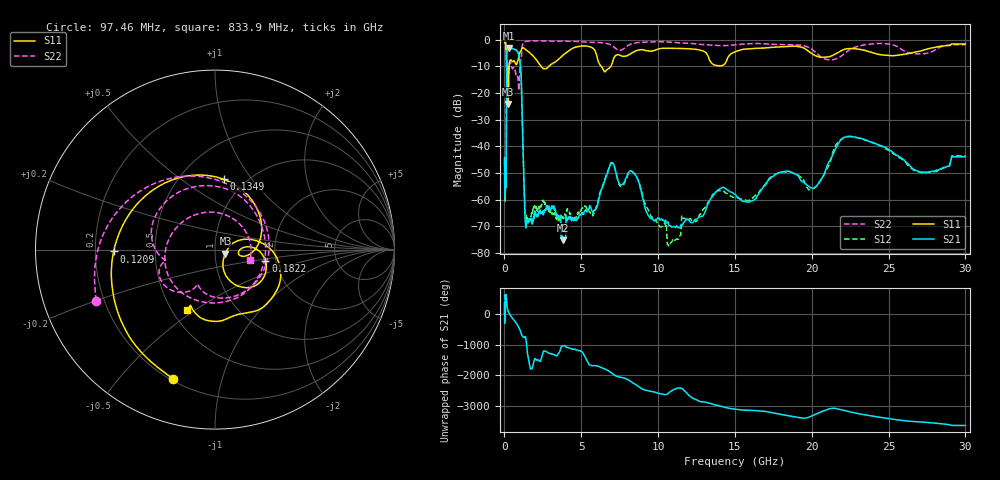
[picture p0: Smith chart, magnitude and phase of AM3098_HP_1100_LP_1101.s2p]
! Date/Time: Thu, Feb 28, 2019 8:44 AM
! Network Analyzer: Agilent Technologies E8364B Rev: A.07.50.67
! Sweep from 0.010 to 30.000 GHz, 1601 Points, Sweep Type: LOG
! Power Supply: 5.022 V, 0.002 A
# Hz S DB R 50
!freq MagS11 AngS11 MagS21 AngS21 MagS12 AngS12 MagS22 AngS22
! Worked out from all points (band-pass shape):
!   1601 points, 10 MHz to 30 GHz, reference 50 ohm
!   highest |S21| = -3.10 dB at 266.5 MHz (marker M1); lowest = -75.4 dB at 3.817 GHz (marker M2)
!   |S21| within 3 dB of the highest: 149.2 MHz to 943.7 MHz (794.5 MHz wide, 145 % of centre)
!   lowest |S11| = -24.1 dB at 248.4 MHz (marker M3), VSWR 1.13, Z = 56.1 - j2.53 ohm
!   |S11| at or under -10 dB: 140.1 MHz to 310.6 MHz (170.5 MHz wide, 75.6 % of centre); 2.372 GHz to 2.907 GHz (534.3 MHz wide, 20.2 % of centre); 6.291 GHz to 6.926 GHz (634.8 MHz wide, 9.61 % of centre)
!   |S22| runs from -19.1 to -0.4 dB; largest |S21 - S12| = 0.011
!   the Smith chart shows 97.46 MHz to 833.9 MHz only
!   S11 on the Smith chart (normalised r, x): 97.46 MHz: 0.21, -0.71; 120.9 MHz: 0.28, -0.01; 134.9 MHz: 0.80, +0.74; 182.2 MHz: 1.76, -0.23; 833.9 MHz: 0.59, -0.46
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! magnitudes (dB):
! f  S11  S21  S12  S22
! 10 MHz  -0.3  -46.6  -44.1  -0.6
! 38.04 MHz  -0.4  -57.1  -55.2  -0.9
! 97.46 MHz  -2.4  -54.4  -52.7  -2.9
! 120.9 MHz  -5.0  -36.3  -35.7  -6.4
! 134.9 MHz  -8.1  -14.7  -14.7  -10.5
! 144.7 MHz  -12.3  -7.5  -7.4  -11.7
! 182.2 MHz  -10.8  -3.9  -3.9  -9.8
! 248.4 MHz  -24.1  -3.1  -3.1  -11.0
! 266.5 MHz  -17.9  -3.1  -3.1  -10.7
! 550.5 MHz  -8.2  -3.5  -3.4  -10.8
! 833.9 MHz  -8.6  -4.4  -4.4  -13.9
! 1.071 GHz  -4.3  -12.0  -12.0  -7.7
! 1.375 GHz  -3.7  -69.9  -66.2  -0.7
! 2.084 GHz  -7.6  -66.0  -63.6  -0.5
! 3.172 GHz  -8.9  -62.8  -65.5  -0.6
! 3.817 GHz  -5.8  -75.4  -66.8  -0.5
! 7.926 GHz  -6.1  -51.7  -52.4  -2.7
! 11.03 GHz  -3.3  -70.1  -75.3  -1.1
! 13.81 GHz  -9.7  -57.1  -56.9  -2.2
! 20.1 GHz  -5.6  -55.8  -55.9  -4.0
! 22.44 GHz  -3.4  -36.4  -36.3  -3.9
! 30 GHz  -1.6  -43.9  -43.7  -1.9
